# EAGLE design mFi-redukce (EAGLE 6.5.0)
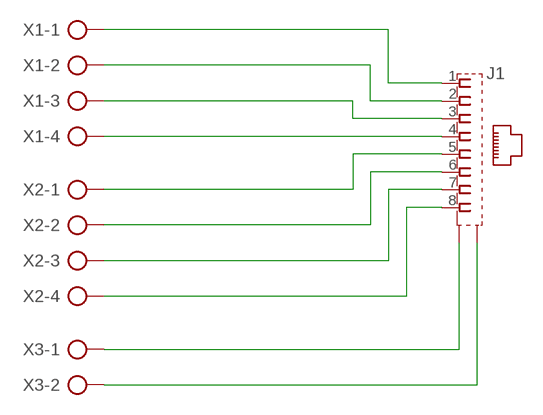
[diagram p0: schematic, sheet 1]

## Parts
J1  555153-1  [555153-1]
X1  AK500/4  [AK500/4]
X2  AK500/4  [AK500/4]
X3  AK500/2  [AK500/2]

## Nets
N$1: J1.1 X1.1
N$2: J1.2 X1.2
N$3: J1.3 X1.3
N$4: J1.4 X1.4
N$5: J1.5 X2.1
N$6: J1.6 X2.2
N$7: J1.7 X2.3
N$8: J1.8 X2.4
N$17: J1.G1(S1) X3.1
N$18: J1.G2(S2) X3.2

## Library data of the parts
J1 = con-amp:555153-1: AMP connector
X1 X2 = con-ptr500:AK500/4: CONNECTOR; OC_FARNELL: unknown; OC_NEWARK: unknown
X3 = con-ptr500:AK500/2: CONNECTOR; OC_FARNELL: unknown; OC_NEWARK: unknown

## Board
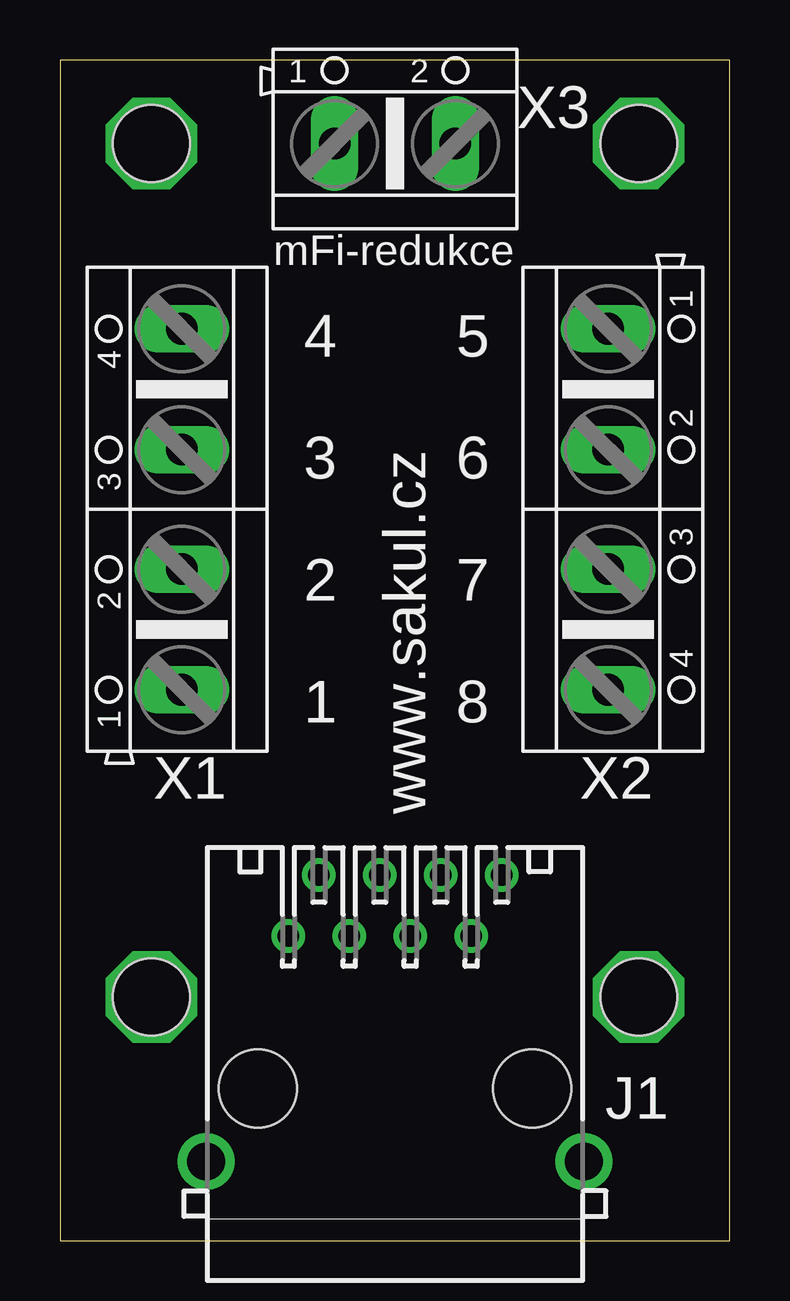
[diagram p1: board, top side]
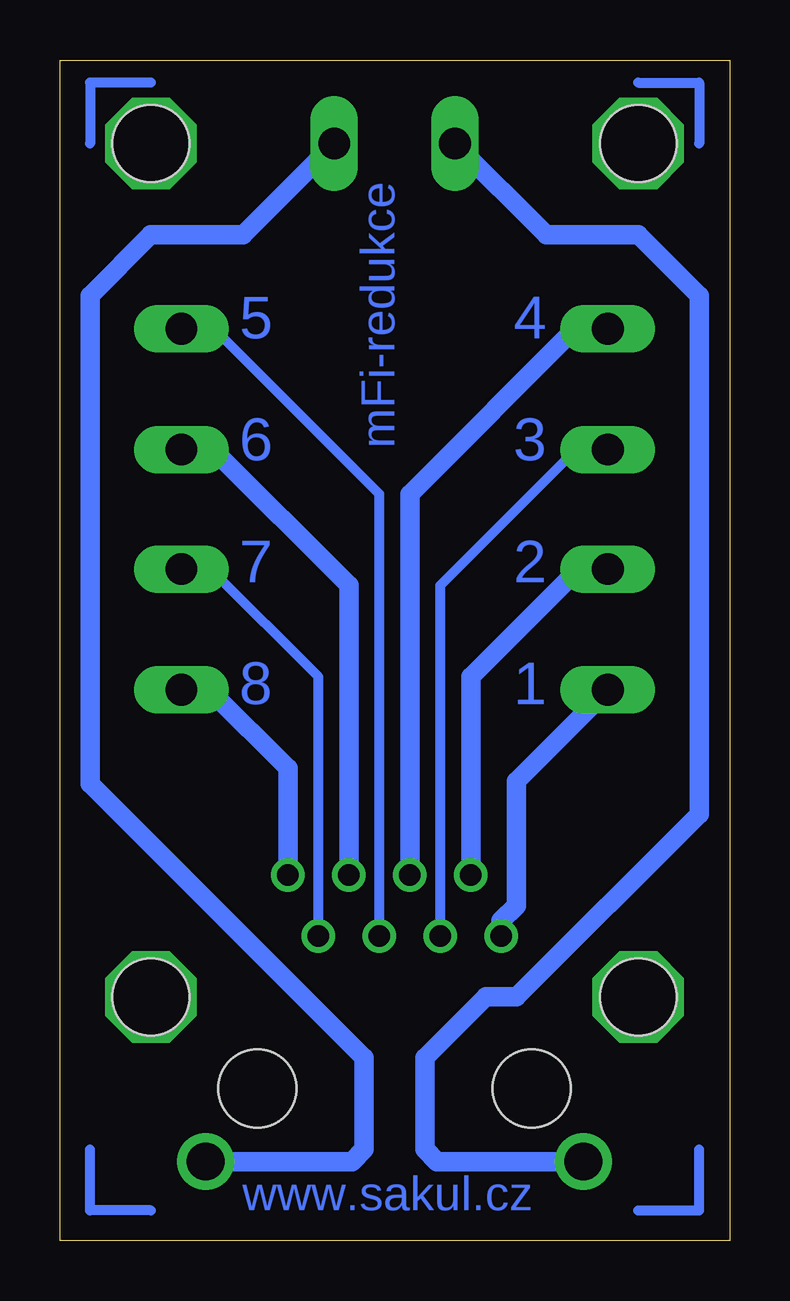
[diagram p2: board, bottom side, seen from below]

Size 27.92 x 49.2 mm. Coordinates in mm from the lower left corner, seen from the top.
Outline: 0,0 27.92,0 27.92,49.2 0,49.2 0,0
Copper layers (1*16): Top 0.035mm / dielectric 1.5mm / Bottom 0.035mm
Design rules "default": minimum track width 10mil, minimum drill 24mil, track to track 8mil, track to pad 8mil, pad to pad 8mil, via to via 8mil, smd to smd 8mil, copper to edge 40mil, drill to drill 8mil, minimum pad ring 10mil, minimum via ring 8mil, stop-mask expansion 4mil, vias tented up to drill 0mil, thermal gap 10mil
Holes 3.2 mm at 3.81,45.72 24.13,45.72 24.13,10.16 3.81,10.16

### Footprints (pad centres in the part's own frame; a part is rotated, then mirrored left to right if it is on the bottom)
555153-1 = drill 0.889: 1 -4.445,6.35; 2 -3.175,8.89; 3 -1.905,6.35; 4 -0.635,8.89; 5 0.635,6.35; 6 1.905,8.89; 7 3.175,6.35; 8 4.445,8.89 | drill 1.575 pad 2.184: G1 -7.874,-3.048; G2 7.874,-3.048 | hole 3.251: -5.715,0; 5.715,0
AK500/4 = drill 1.321 long: 1 -7.518,0; 2 -2.489,0; 3 2.489,0; 4 7.518,0
AK500/2 = drill 1.321 long: 1 -2.515,0; 2 2.515,0

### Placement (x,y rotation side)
J1  13.97,6.35 0 top
X1  5.08,30.48 90 top
X2  22.86,30.48 270 top
X3  13.97,45.72 0 top

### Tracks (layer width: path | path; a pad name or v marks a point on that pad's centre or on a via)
N$1
  Bottom 0.813: J1.1 9.53,13.34 8.89,13.97 8.89,19.15 X1.1
N$2
  Bottom 0.813: J1.2 10.79,23.5 6.35,27.94 6.4,27.94 X1.2
N$3
  Bottom 0.406: J1.3 12.06,27.3 6.35,33.02 5.13,33.02 X1.3
N$4
  Bottom 0.813: J1.4 13.34,31.11 6.35,38.1 6.45,38.1 X1.4
N$5
  Bottom 0.406: J1.5 14.61,31.11 21.59,38.1 21.49,38.1 X2.1
N$6
  Bottom 0.813: X2.2 21.54,32.97 15.88,27.3 J1.6
N$7
  Bottom 0.406: J1.7 17.14,23.5 21.59,27.94 21.54,27.94 X2.3
N$8
  Bottom 0.813: J1.8 18.41,19.68 21.59,22.86 21.49,22.86 X2.4
N$9  (via drill 0.6 pad 3.81)
  other vias: 3.81,45.72
N$10  (via drill 0.6 pad 3.81)
  other vias: 24.13,45.72
N$11  (via drill 0.6 pad 3.81)
  other vias: 24.13,10.16
N$12  (via drill 0.6 pad 3.81)
  other vias: 3.81,10.16
N$13
  Bottom 0.406: 3.81,1.27 1.27,1.27 1.27,3.81
N$14
  Bottom 0.406: 24.13,1.27 26.67,1.27 26.67,3.81
N$15
  Bottom 0.406: 3.81,48.26 1.27,48.26 1.27,45.72
N$16
  Bottom 0.406: 24.13,48.26 26.67,48.26 26.67,45.72
N$17
  Bottom 0.813: J1.G1 12.19,3.3 12.7,3.81 12.7,7.62 10.16,10.16 8.89,10.16 1.27,17.78 1.27,39.37 3.81,41.91 7.64,41.91 X3.1
N$18
  Bottom 0.813: J1.G2 15.75,3.3 15.24,3.81 15.24,7.62 26.67,19.05 26.67,39.37 24.13,41.91 20.3,41.91 X3.2

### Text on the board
Bottom: 4 | 5 | 3 | 6 | mFi-redukce | 2 | 7 | 1 | 8 | www.sakul.cz
tPlace: mFi-redukce | 4 | 5 | 3 | 6 | 2 | 7 | 1 | 8 | www.sakul.cz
